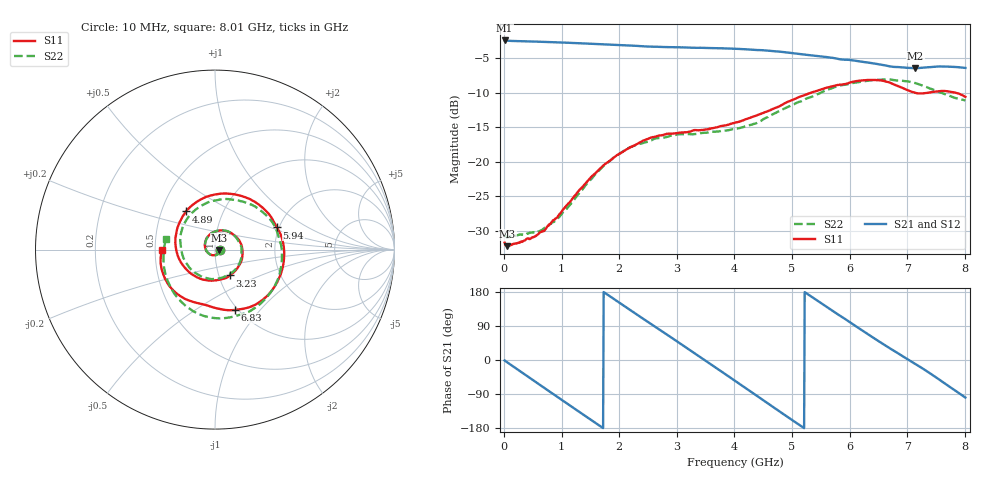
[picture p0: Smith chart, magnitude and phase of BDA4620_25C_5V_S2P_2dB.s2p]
!Agilent Technologies,E5071B,MY42404982,A.09.10
!Date: Wed May 06 08:58:30 2026
!Data & Calibration Information:
!Freq	S11:SOLT2(ON)	S21:SOLT2(ON)	S12:SOLT2(ON)	S22:SOLT2(ON)
# Hz S RI R 50
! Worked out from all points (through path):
!   801 points, 10 MHz to 8.01 GHz, reference 50 ohm
!   highest |S21| = -2.44 dB at 10 MHz (marker M1); lowest = -6.5 dB at 7.14 GHz (marker M2)
!   group delay of S21, straight-line fit = 284 ps
!   lowest |S11| = -32.2 dB at 60 MHz (marker M3), VSWR 1.05, Z = 52.5 - j0.4 ohm
!   |S11| at or under -10 dB: start of sweep to 5.328 GHz; 7.132 GHz to 7.368 GHz (236.2 MHz wide, 3.26 % of centre); 7.837 GHz to end of sweep
!   |S22| runs from -31.0 to -8.1 dB; largest |S21 - S12| = 0.0033
!   S11 on the Smith chart (normalised r, x): 10 MHz: 1.05, -0.00; 3.23 GHz: 1.13, -0.33; 4.89 GHz: 0.67, +0.30; 5.94 GHz: 1.95, +0.55; 6.83 GHz: 0.97, -0.75; 8.01 GHz: 0.54, -0.00
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1e7  0.0259 -0.00189  0.7546 -0.016  0.7556 -0.0162  0.0296 -0.00194
6e7  0.0243 -0.00381  0.7466 -0.0862  0.7482 -0.0875  0.0282 -0.00364
3.7e8  0.0178 -0.0206  0.5767 -0.4697  0.5769 -0.4713  0.0214 -0.0211
7.3e8  -0.0106 -0.0313  0.1673 -0.7166  0.1668 -0.7178  -0.00712 -0.0331
1.03e9  -0.0431 -0.0145  -0.2267 -0.6921  -0.2276 -0.693  -0.0401 -0.0169
1.35e9  -0.0566 0.0325  -0.5628 -0.4489  -0.5633 -0.4492  -0.0553 0.0292
1.93e9  0.0243 0.1066  -0.6532 0.2545  -0.6541 0.2555  0.0213 0.1071
2.32e9  0.1112 0.0771  -0.3293 0.605  -0.3303 0.6062  0.1086 0.0783
2.68e9  0.1542 -0.0101  0.0939 0.6721  0.0945 0.6732  0.1485 -0.000947
3.23e9  0.0818 -0.144  0.6031 0.2912  0.6043 0.2908  0.088 -0.132
3.61e9  -0.0272 -0.1726  0.6467 -0.1522  0.648 -0.1531  -0.0189 -0.1643
4.01e9  -0.1478 -0.1221  0.378 -0.5375  0.3779 -0.5381  -0.136 -0.1074
4.44e9  -0.2196 0.023  -0.1075 -0.6337  -0.1091 -0.6341  -0.1921 0.0361
4.89e9  -0.1619 0.2127  -0.5194 -0.3389  -0.5197 -0.3396  -0.1141 0.2174
5.35e9  0.061 0.3129  -0.5703 0.1434  -0.5707 0.1442  0.1047 0.2773
5.94e9  0.3452 0.1232  -0.1551 0.5254  -0.1544 0.5266  0.3547 0.0709
6.3e9  0.373 -0.1158  0.18 0.4918  0.1818 0.4923  0.3567 -0.146
6.68e9  0.2029 -0.3169  0.415 0.2641  0.4163 0.2644  0.2061 -0.3361
6.83e9  0.1114 -0.3365  0.459 0.1553  0.4605 0.1551  0.1153 -0.3694
7.14e9  -0.0368 -0.3135  0.4678 -0.0863  0.4688 -0.0874  -0.0858 -0.3616
7.63e9  -0.2429 -0.2167  0.2481 -0.4216  0.2485 -0.4226  -0.2718 -0.1525
8.01e9  -0.2955 -0.00347  -0.0756 -0.4717  -0.0761 -0.4728  -0.2713 0.0589
